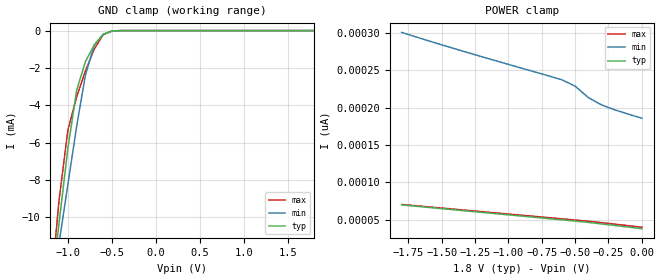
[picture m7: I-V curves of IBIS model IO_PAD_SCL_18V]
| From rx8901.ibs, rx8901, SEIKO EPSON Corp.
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[Model]   IO_PAD_SCL_18V
Model_type Input
Polarity Non-Inverting
Vinh=1.26
Vinl=0.54
C_comp   2.5p   2.0p   3.0p
[Temperature Range] 25   105   -40
[Voltage Range]   1.80   1.60   2.00
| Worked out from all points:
|   GND clamp passes 1 mA (typ) near -0.73 V on its own axis
[GND Clamp]
-1.8V     -38.99mA   -33.75mA   -45.17mA
-1.2V     -14.34mA   -14.53mA   -14.15mA
-1.1V     -10.29mA   -11.38mA   -9.067mA
-1V       -6.296mA   -8.231mA   -5.323mA
-900mV    -3.187mA   -5.113mA   -3.55mA
-800mV    -1.654mA   -2.365mA   -2.158mA
-700mV    -763.9uA   -779.4uA   -983.1uA
-600mV    -207.7uA   -205uA     -228.8uA
-500mV    -21.87uA   -34.9uA    -13.49uA
-400mV    -1.211uA   -3.926uA   -277.5nA
1.8V      38.08pA    197pA      35.91pA
[POWER Clamp]
-1.8V     69.91pA    300.8pA    70.49pA
-1.3V     61.57pA    273.6pA    62.48pA
-600mV    49.94pA    237.5pA    51.27pA
-500mV    48.28pA    229pA      49.67pA
-400mV    46.46pA    213.6pA    48.04pA
-300mV    44.39pA    203.6pA    46.15pA
-200mV    42.29pA    197pA      44.11pA
0V        38.08pA    186pA      40.01pA
